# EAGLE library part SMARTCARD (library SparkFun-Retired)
Smart card socket- PRT-09368
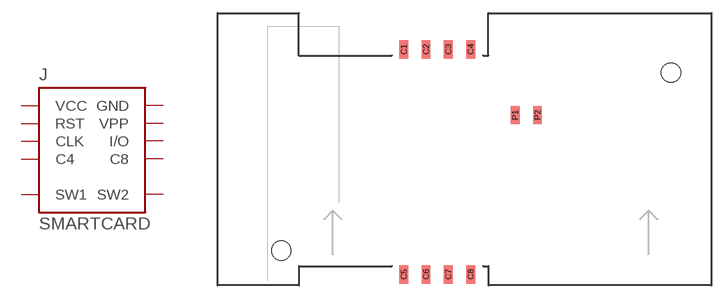
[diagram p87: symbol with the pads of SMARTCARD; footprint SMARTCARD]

Designator prefix J

## SMARTCARDSMD  [SMARTCARD]
C1  VCC
C2  RST
C3  CLK
C4  C4
C5  GND
C6  VPP
C7  I/O
C8  C8
P1  SW1
P2  SW2

## Footprint SMARTCARD (pad centres in mm)
Description: S..m..r..t. I am so smrt!
smd 1 x 2.1: C1 -6.92,11.4; C2 -4.38,11.4; C3 -1.84,11.4; C4 0.7,11.4; C5 -6.92,-14.3; C6 -4.38,-14.3; C7 -1.84,-14.3; C8 0.7,-14.3; P1 5.78,3.91; P2 8.32,3.91
hole 2.2 at 23.56,8.75
hole 2.2 at -20.89,-11.57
